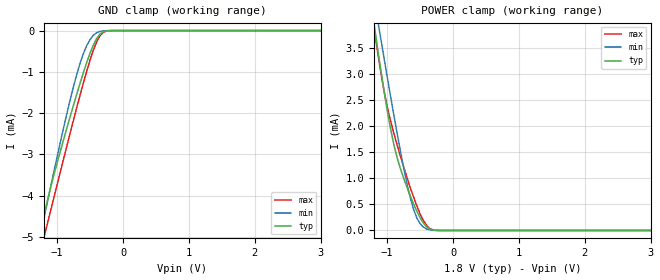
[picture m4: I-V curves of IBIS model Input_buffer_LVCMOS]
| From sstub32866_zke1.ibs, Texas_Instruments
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[Model]   Input_buffer_LVCMOS
Model_type   Input
Polarity   Non-Inverting
Vinl   =   0.650V
Vinh   =   1.150V
|Variable   typ   min   max
C_comp   3.761e-13   2.569e-13   4.547e-13
|Variable   typ   min   max
[Voltage range]   1.8   1.7   1.9
|Variable   typ   min   max
[Temperature range]  27   125   0.0
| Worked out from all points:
|   GND clamp passes 1 mA (typ) near -0.60 V on its own axis
|   POWER clamp passes 1 mA (typ) near -0.75 V on its own axis
[GND_clamp]
|Volts   typ   min   max
-3.6V     -26.93mA   -23.68mA   -28.13mA
-1.25V    -4.843mA   -4.929mA   -5.339mA
-1.2V     -4.474mA   -4.547mA   -5.012mA
-1.15V    -4.128mA   -4.168mA   -4.688mA
-900mV    -2.627mA   -2.336mA   -3.092mA
-700mV    -1.524mA   -1.045mA   -1.848mA
-550mV    -766.6uA   -359.9uA   -976uA
-500mV    -544uA     -214.5uA   -712uA
-400mV    -190.8uA   -50.47uA   -272.1uA
-300mV    -28.64uA   -6.757uA   -43.37uA
-200mV    -1.7uA     -615.2nA   -2.123uA
3.6V      0A         0A         0A
[POWER_clamp]
|Volts   typ   min   max
-3.6V     26.84mA    23.61mA    28.03mA
-1.2V     3.957mA    4.453mA    3.885mA
-1.15V    3.522mA    4.072mA    3.455mA
-1.1V     3.098mA    3.693mA    3.051mA
-950mV    1.954mA    2.579mA    2.104mA
-850mV    1.399mA    1.867mA    1.642mA
-700mV    825.8uA    898.4uA    1.017mA
-600mV    508.2uA    405.4uA    640.4uA
-500mV    244uA      130.3uA    318.2uA
-400mV    68.76uA    27.15uA    92.99uA
-200mV    370.5nA    280.8nA    343.2nA
3.6V      0A         0A         0A
